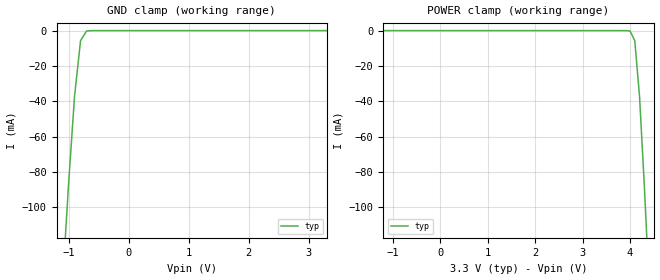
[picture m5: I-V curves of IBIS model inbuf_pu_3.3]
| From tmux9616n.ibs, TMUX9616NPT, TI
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| inbuf_pu_3.3
[Model]   inbuf_pu_3.3
Model_type   Input
Vinl = 0.99
Vinh = 1.98
|   typ   min   max
C_comp   1.008417e-12   NA   NA
[Voltage Range]   3.3   NA   NA
[Temperature Range]   27   NA   NA
[Power Clamp Reference]   3.3   NA   NA
[GND Clamp Reference]   0   NA   NA
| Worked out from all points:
|   GND clamp passes 1 mA (typ) near -0.71 V on its own axis
[GND Clamp]
|   Voltage   I(typ)   I(min)   I(max)
-6.6V     -3.715A    NA         NA
-1.1V     -143.3mA   NA         NA
-1V       -86.97mA   NA         NA
-900mV    -37.12mA   NA         NA
-800mV    -5.701mA   NA         NA
-700mV    -221.4uA   NA         NA
3.3V      24pA       NA         NA
[POWER Clamp]
|   Voltage   I(typ)   I(min)   I(max)
-3.3V     84.69pA    NA         NA
4V        -221.4uA   NA         NA
4.1V      -5.701mA   NA         NA
4.2V      -37.12mA   NA         NA
4.3V      -86.97mA   NA         NA
4.4V      -143.3mA   NA         NA
6.6V      -1.549A    NA         NA
